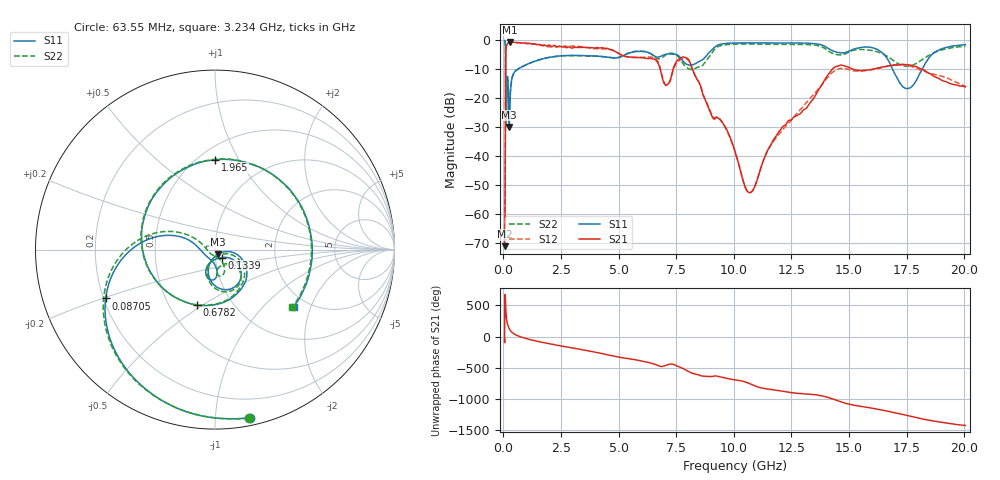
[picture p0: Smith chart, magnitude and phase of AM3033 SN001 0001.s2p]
# Hz S DB R 50
!freq MagS11 AngS11 MagS21 AngS21 MagS12 AngS12 MagS22 AngS22
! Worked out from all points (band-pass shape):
!   1601 points, 50 MHz to 20.05 GHz, reference 50 ohm
!   highest |S21| = -0.68 dB at 295.2 MHz (marker M1); lowest = -71.1 dB at 54.3 MHz (marker M2)
!   |S21| within 3 dB of the highest: 105.6 MHz to 4.781 GHz (4.676 GHz wide, 191 % of centre)
!   lowest |S11| = -30.0 dB at 249.4 MHz (marker M3), VSWR 1.07, Z = 51.6 - j2.77 ohm
!   |S11| at or under -10 dB: 92.48 MHz to 629 MHz (536.6 MHz wide, 149 % of centre); 16.89 GHz to 18.18 GHz (1.294 GHz wide, 7.38 % of centre)
!   |S22| runs from -29.7 to -0.1 dB; largest |S21 - S12| = 0.062
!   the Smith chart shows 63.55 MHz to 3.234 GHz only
!   S11 on the Smith chart (normalised r, x): 63.55 MHz: 0.06, -1.23; 87.05 MHz: 0.21, -0.20; 133.9 MHz: 1.08, -0.10; 678.2 MHz: 0.68, -0.47; 1.965 GHz: 0.60, +0.80; 3.234 GHz: 1.69, -1.53
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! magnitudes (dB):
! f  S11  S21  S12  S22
! 50 MHz  -0.2  -66.5  -65.3  -0.1
! 54.3 MHz  -0.2  -71.1  -64.4  -0.2
! 63.55 MHz  -0.4  -67.8  -66.7  -0.4
! 87.05 MHz  -3.5  -19.5  -19.5  -3.6
! 100.7 MHz  -23.7  -4.7  -4.7  -29.7
! 133.9 MHz  -24.6  -1.8  -1.8  -19.7
! 135.9 MHz  -22.9  -1.8  -1.8  -18.8
! 179.4 MHz  -12.9  -1.3  -1.3  -12.5
! 249.4 MHz  -30.0  -0.7  -0.7  -28.3
! 295.2 MHz  -18.5  -0.7  -0.7  -18.7
! 369.6 MHz  -13.1  -0.8  -0.7  -13.3
! 678.2 MHz  -9.7  -0.9  -0.9  -9.8
! 1.005 GHz  -8.5  -1.3  -1.1  -8.5
! 1.965 GHz  -6.0  -1.7  -2.3  -6.0
! 2.722 GHz  -5.3  -2.6  -2.2  -5.4
! 3.234 GHz  -5.3  -2.6  -2.2  -5.4
! 7.402 GHz  -4.9  -9.0  -9.7  -4.7
! 8.129 GHz  -8.6  -8.4  -8.5  -10.1
! 10.69 GHz  -1.0  -52.6  -52.6  -1.4
! 14.47 GHz  -4.2  -9.0  -10.2  -5.0
! 17.52 GHz  -16.7  -8.5  -8.6  -9.1
! 20.05 GHz  -1.6  -16.1  -15.9  -2.2
